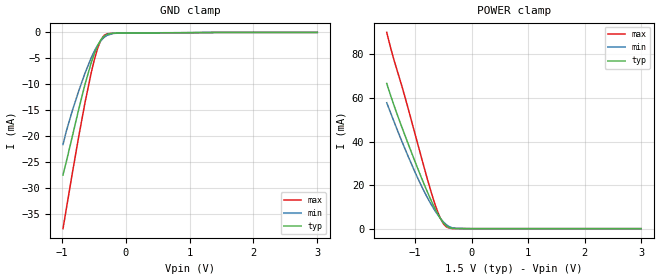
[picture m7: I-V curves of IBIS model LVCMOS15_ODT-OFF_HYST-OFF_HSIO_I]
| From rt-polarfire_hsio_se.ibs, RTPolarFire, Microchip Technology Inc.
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|   Model LVCMOS15_ODT-OFF_HYST-OFF_HSIO_I
[Model]   LVCMOS15_ODT-OFF_HYST-OFF_HSIO_I
Model_type   Input
Vinl =   0.525
Vinh =   0.975
|   typ   min   max
C_comp_pullup   1.335e-12   1.335e-12   1.380e-12
C_comp_pulldown  1.335e-12   1.335e-12   1.380e-12
[Temperature Range]  25C   125C   -55C
[Voltage Range]  1.5   1.425   1.575
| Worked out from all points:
|   GND clamp passes 1 mA (typ) near -0.36 V on its own axis
|   POWER clamp passes 1 mA (typ) near -0.43 V on its own axis
[GND Clamp]
| Voltage   I(typ)   I(min)   I(max)
-984.4mV  -27.52mA   -21.64mA   -37.88mA
-935.2mV  -25.11mA   -19.19mA   -34.26mA
-836.7mV  -19.99mA   -15.05mA   -27.09mA
-738.3mV  -14.86mA   -11.32mA   -20.13mA
-639.8mV  -10.04mA   -7.878mA   -13.59mA
-541.4mV  -5.828mA   -4.867mA   -7.743mA
-443mV    -2.601mA   -2.515mA   -3.122mA
-393.7mV  -1.488mA   -1.649mA   -1.54mA
-344.5mV  -752.5uA   -1.007mA   -611.2uA
-196.9mV  -143.7uA   -195uA     -157.5uA
-49.22mV  -115.8uA   -100.4uA   -145.1uA
3V        0A         0A         0A
[POWER Clamp]
| Voltage   I(typ)   I(min)   I(max)
-1.5V     66.68mA    57.83mA    90.15mA
-1.378V   57.1mA     49.63mA    78.06mA
-1.28V    49.95mA    43.17mA    69.59mA
-984.4mV  29.77mA    25.04mA    42.07mA
-836.7mV  20.27mA    17.03mA    27.95mA
-689.1mV  11.54mA    10.05mA    14.67mA
-590.6mV  6.461mA    6.118mA    7.191mA
-541.4mV  4.305mA    4.424mA    4.25mA
-443mV    1.22mA     1.775mA    783.3uA
-344.5mV  141uA      412.1uA    66.01uA
-49.22mV  6.174uA    9.105uA    8.248uA
3V        0A         0A         0A
